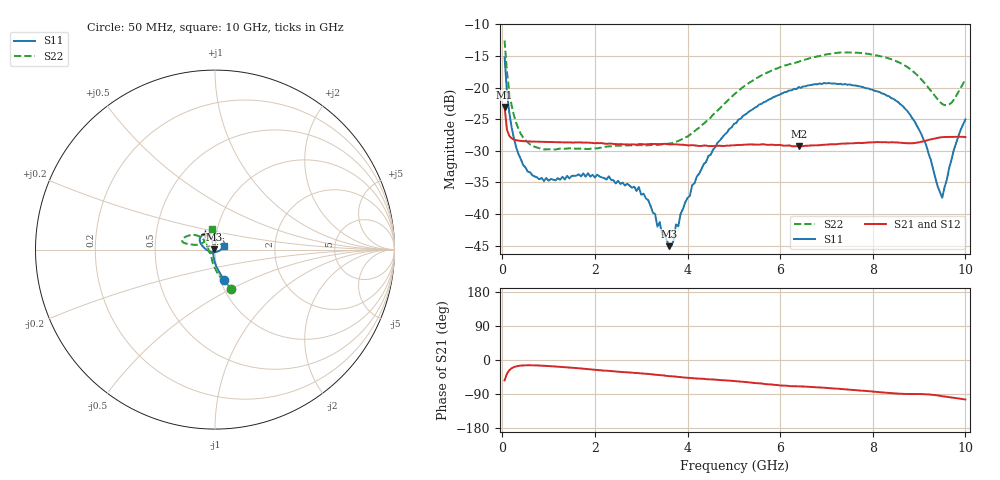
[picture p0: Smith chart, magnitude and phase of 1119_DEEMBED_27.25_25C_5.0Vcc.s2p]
!Hittite Microwave Corp.
!Digital Attenuator/PhaseShifter Rev 1.4.0
!Filename: C:\DATA\DATA\1119_DEEMBED_27.25_25C_5.0Vcc.s2p
!VNA ID: Agilent Technologies,N5224A,MY51441122,A.10.45.03
!Device type:
!2 Port Calibration.
!Temp(C): 25
!Lot Number:
!Serial Number:
!Operator:
!Misc:
!Attenuator:  27.250
# GHZ S DB R 50.0
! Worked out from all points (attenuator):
!   200 points, 50 MHz to 10 GHz, reference 50 ohm
!   highest |S21| = -23.08 dB at 50 MHz (marker M1); lowest = -29.3 dB at 6.4 GHz (marker M2)
!   lowest |S11| = -45.1 dB at 3.6 GHz (marker M3), VSWR 1.01, Z = 49.5 + j0.154 ohm
!   |S11| at or under -10 dB: start of sweep to end of sweep
!   |S22| runs from -29.8 to -12.6 dB; largest |S21 - S12| = 0.00011
!   S11 on the Smith chart (normalised r, x): 50 MHz: 1.04, -0.36; 6.5 GHz: 0.88, +0.15; 10 GHz: 1.11, +0.05
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0.05  -15.22 -74.1  -23.08 -53.7  -23.08 -53.7  -12.56 -67.4
0.1  -20.66 -86.2  -26.65 -36.6  -26.65 -36.6  -17.51 -83.9
0.2  -26.23 -97.8  -28.01 -21.9  -28.03 -21.9  -22.78 -100.6
0.45  -32.23 -114.2  -28.46 -14.3  -28.47 -14.3  -27.88 -121.3
0.9  -34.78 -130.7  -28.59 -15.2  -28.59 -15.3  -29.77 -135.8
1.75  -33.57 -136.7  -28.70 -23.0  -28.71 -23.0  -29.66 -140.7
2.95  -35.72 -126.7  -28.94 -34.6  -28.96 -34.7  -29.12 -160.0
3.3  -40.02 -142.7  -28.92 -38.7  -28.94 -38.8  -29.05 -170.5
3.35  -41.99 -139.9  -28.94 -39.3  -28.96 -39.3  -29.09 -172.1
3.4  -41.26 -151.4  -28.93 -39.7  -28.94 -39.7  -29.03 -173.6
3.45  -43.24 -160.1  -28.93 -40.4  -28.94 -40.4  -28.96 -175.4
3.6  -45.07 163.8  -28.98 -42.5  -28.98 -42.6  -28.87 178.9
4.2  -34.06 98.2  -29.19 -48.8  -29.21 -48.8  -26.60 154.1
5.05  -25.61 100.7  -29.10 -55.8  -29.12 -55.9  -20.83 138.7
6.4  -19.93 121.2  -29.30 -69.6  -29.32 -69.6  -15.93 149.9
6.5  -19.81 123.0  -29.26 -69.8  -29.28 -69.8  -15.67 151.4
6.7  -19.56 126.8  -29.14 -71.4  -29.16 -71.4  -15.25 153.9
8.35  -21.37 157.4  -28.67 -86.9  -28.67 -86.9  -15.41 168.1
8.999999  -26.66 -177.6  -28.65 -89.7  -28.65 -89.7  -18.35 167.4
9.5  -37.42 -71.9  -27.85 -95.4  -27.86 -95.5  -22.62 144.0
9.75  -29.86 -0.7  -27.80 -99.7  -27.81 -99.7  -21.93 114.2
10  -25.04 24.0  -27.84 -104.2  -27.83 -104.1  -18.68 98.5
